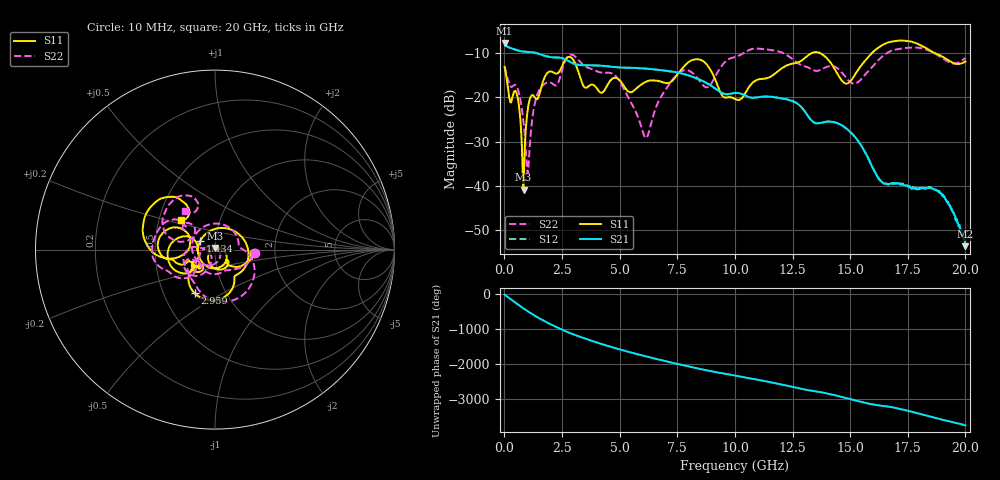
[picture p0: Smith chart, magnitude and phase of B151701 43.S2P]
!  2-Port S-parameters saved by WinCal
! VAR MeasName=S-Parameters (CALIBRATED_DATA) read from VNA (N5244A)
! VAR MeasDate=2015-12-24 19:14:30
! VAR NAME=B151701 43
! VAR FILENAME=B151701 43.S2P
! VAR DATE=2015-12-24 19:14:30
! VAR PHYS_PORTS=1,3
# Hz S DB R 50
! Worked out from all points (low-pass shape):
!   801 points, 10 MHz to 20 GHz, reference 50 ohm
!   highest |S21| = -7.85 dB at 10 MHz (marker M1); lowest = -53.5 dB at 20 GHz (marker M2)
!   |S21| within 3 dB of the highest: start of sweep to 1.84 GHz
!   lowest |S11| = -40.8 dB at 834.6 MHz (marker M3), VSWR 1.02, Z = 50.2 + j0.882 ohm
!   |S11| at or under -10 dB: start of sweep to 13.38 GHz; 13.64 GHz to 15.97 GHz (2.325 GHz wide, 15.7 % of centre); 18.63 GHz to end of sweep
!   |S22| runs from -37.2 to -8.9 dB; largest |S21 - S12| = 0.0013
!   S11 on the Smith chart (normalised r, x): 10 MHz: 1.55, -0.07; 1.434 GHz: 0.84, +0.08; 2.959 GHz: 0.72, -0.38; 20 GHz: 0.65, +0.22
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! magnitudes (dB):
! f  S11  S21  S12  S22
! 10 MHz  -13.3  -7.8  -7.9  -13.1
! 259.9 MHz  -21.2  -8.9  -8.9  -17.5
! 559.7 MHz  -19.7  -9.5  -9.5  -17.9
! 834.6 MHz  -40.8  -9.8  -9.8  -25.9
! 1.034 GHz  -22.1  -9.9  -9.8  -36.4
! 1.434 GHz  -20.4  -10.2  -10.2  -19.3
! 1.859 GHz  -14.6  -10.9  -10.9  -16.7
! 2.959 GHz  -11.4  -12.4  -12.4  -10.5
! 3.358 GHz  -16.6  -12.8  -12.8  -12.5
! 4.208 GHz  -19.0  -12.9  -12.9  -14.5
! 4.858 GHz  -15.7  -13.3  -13.3  -15.4
! 6.132 GHz  -16.6  -13.6  -13.6  -29.2
! 6.682 GHz  -16.4  -13.9  -13.9  -21.0
! 7.681 GHz  -13.8  -14.7  -14.7  -14.2
! 8.456 GHz  -11.6  -16.0  -16.1  -16.2
! 10.01 GHz  -20.4  -19.1  -19.1  -11.0
! 12.43 GHz  -12.6  -20.8  -20.7  -11.2
! 13.35 GHz  -10.1  -25.4  -25.4  -13.8
! 14.85 GHz  -17.0  -27.2  -27.1  -15.8
! 16.68 GHz  -7.7  -39.6  -39.5  -9.9
! 18.85 GHz  -10.5  -41.4  -41.1  -10.8
! 20 GHz  -12.0  -53.5  -52.7  -11.2
